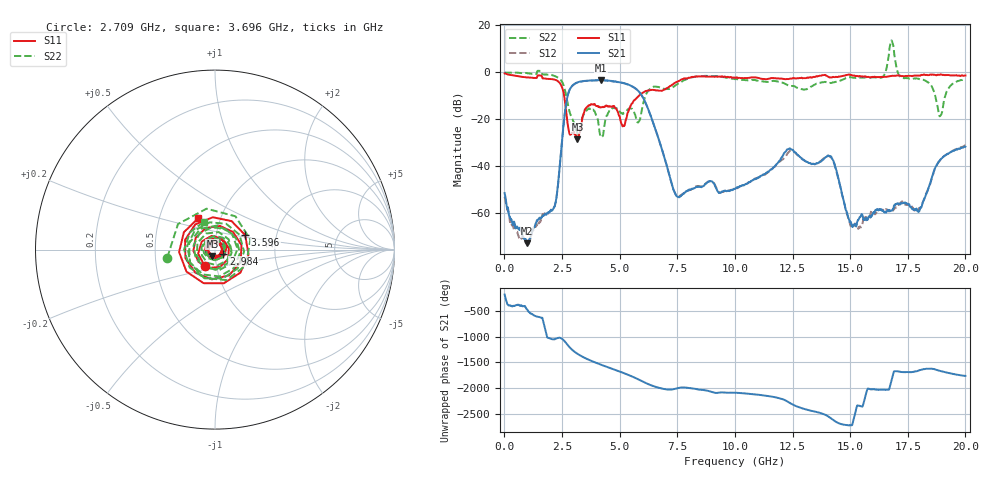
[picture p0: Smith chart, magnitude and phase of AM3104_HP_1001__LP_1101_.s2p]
!Created with skrf (http://scikit-rf.org).
# Hz S RI R 50.0
!freq ReS11 ImS11 ReS21 ImS21 ReS12 ImS12 ReS22 ImS22
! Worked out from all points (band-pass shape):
!   1601 points, 10 MHz to 20 GHz, reference 50 ohm
!   highest |S21| = -3.25 dB at 4.183 GHz (marker M1); lowest = -72.7 dB at 984.5 MHz (marker M2)
!   |S21| within 3 dB of the highest: 2.899 GHz to 5.601 GHz (2.703 GHz wide, 63.6 % of centre)
!   lowest |S11| = -28.4 dB at 3.171 GHz (marker M3), VSWR 1.08, Z = 48.5 - j3.43 ohm
!   |S11| at or under -10 dB: 2.594 GHz to 5.821 GHz (3.227 GHz wide, 76.7 % of centre)
!   |S22| runs from -27.6 to 13.6 dB; largest |S21 - S12| = 0.07
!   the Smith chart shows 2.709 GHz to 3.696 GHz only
!   S11 on the Smith chart (normalised r, x): 2.709 GHz: 0.88, -0.17; 2.984 GHz: 1.10, -0.05; 3.596 GHz: 1.38, +0.23; 3.696 GHz: 0.78, +0.28
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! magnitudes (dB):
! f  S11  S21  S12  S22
! 10 MHz  -0.4  -51.3  -53.0  0.0
! 984.5 MHz  -2.1  -72.7  -73.4  -0.3
! 2.184 GHz  -3.1  -57.0  -56.9  -1.5
! 2.709 GHz  -19.2  -11.6  -11.6  -11.4
! 2.984 GHz  -25.7  -5.3  -5.3  -20.7
! 3.171 GHz  -28.4  -4.3  -4.3  -26.1
! 3.346 GHz  -22.2  -3.8  -3.9  -21.4
! 3.596 GHz  -14.6  -3.5  -3.6  -15.9
! 3.696 GHz  -14.1  -3.4  -3.5  -15.6
! 4.183 GHz  -14.9  -3.2  -3.3  -27.5
! 5.157 GHz  -22.7  -4.5  -4.5  -17.6
! 5.795 GHz  -10.3  -7.7  -7.8  -21.3
! 6.682 GHz  -7.7  -28.0  -28.0  -6.2
! 7.519 GHz  -3.8  -52.9  -52.8  -4.9
! 10.01 GHz  -2.3  -49.6  -49.8  -2.9
! 13.34 GHz  -2.1  -39.0  -39.0  -5.9
! 14.22 GHz  -2.1  -36.6  -36.9  -4.4
! 15.08 GHz  -1.1  -65.0  -65.0  -2.1
! 16.68 GHz  -1.6  -58.6  -59.1  7.3
! 18.01 GHz  -1.4  -58.7  -57.8  -2.9
! 18.9 GHz  -0.9  -37.3  -37.5  -18.6
! 20 GHz  -1.3  -31.6  -31.1  -2.8
